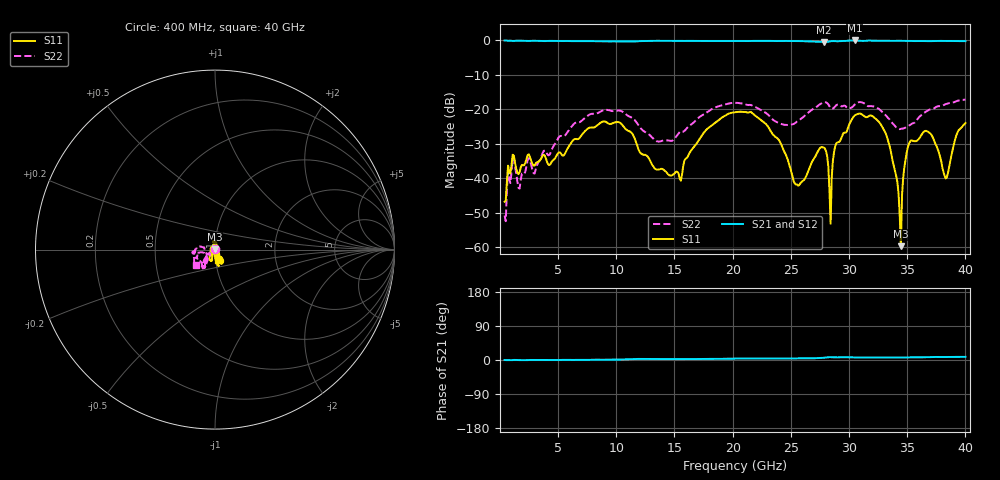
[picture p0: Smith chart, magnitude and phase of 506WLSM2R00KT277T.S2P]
!  American Technical Ceramics  Date:  8/31/2012
!  One Norden Lane
!  Huntington Station,  NY.  11746-2102
!  Tel:  (631) 622-4700  Fax:  (631) 622-4748
!  Part Number  506WLSM2R00KT277T
!  Description:  Ultra-Broadband Inductor
!  Application:  Ultra-broadband DC block decoupling, bias tee
# GHZ S DB R 50
! Freq  |S11|  S11 Ph  |S21|  S21 Ph  |S12|  S12 Ph  |S22|  S22 Ph
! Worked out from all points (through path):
!   401 points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, 400 MHz to 40 GHz, reference 50 ohm
!   highest |S21| = 0.00 dB at 30.5 GHz (marker M1); lowest = -0.5 dB at 27.82 GHz (marker M2)
!   lowest |S11| = -59.7 dB at 34.46 GHz (marker M3), VSWR 1.00, Z = 49.9 + j0.0755 ohm
!   |S11| at or under -10 dB: start of sweep to end of sweep
!   |S22| runs from -52.4 to -17.2 dB; largest |S21 - S12| = 0.0031
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0.4  -46.76 154.5  -0.01 -0.0  -0.01 -0.0  -50.76 132.2
1.192  -33.39 149.7  -0.14 0.2  -0.14 0.2  -34.17 153.8
1.687  -38.20 161.9  -0.06 -0.3  -0.06 -0.3  -42.96 168.4
7.033  -27.40 -110.6  -0.18 0.4  -0.18 0.5  -23.28 -126.0
10.201  -23.70 -115.8  -0.31 1.1  -0.31 1.2  -20.29 -123.8
13.666  -37.43 -140.0  -0.10 2.4  -0.10 2.5  -29.33 -139.6
15.448  -40.08 -137.4  -0.10 2.2  -0.10 2.2  -26.56 -148.8
17.626  -26.30 -88.2  -0.16 2.7  -0.16 2.8  -21.20 -135.6
20.2  -20.79 -78.7  -0.17 3.6  -0.17 3.7  -18.07 -123.6
22.873  -24.27 -80.6  -0.12 4.0  -0.12 4.0  -21.07 -124.0
25.447  -41.80 -91.1  -0.18 4.3  -0.19 4.3  -23.75 -164.1
26.833  -35.08 -123.4  -0.32 4.3  -0.31 4.4  -20.03 -170.0
27.823  -31.03 -149.9  -0.46 5.9  -0.47 5.9  -17.93 -171.4
28.417  -53.17 -19.3  -0.23 7.4  -0.23 7.4  -19.57 -171.7
28.912  -29.81 -65.0  -0.22 6.7  -0.23 6.7  -18.74 -156.4
30.496  -21.73 -56.4  -0.00 6.5  -0.01 6.6  -18.53 -127.9
33.466  -30.36 -78.1  -0.10 6.8  -0.11 6.8  -22.84 -133.7
34.456  -59.65 133.4  -0.10 6.8  -0.10 6.9  -25.63 -159.7
35.248  -29.31 98.3  -0.14 6.9  -0.14 7.0  -24.50 172.3
36.931  -26.82 88.2  -0.19 7.6  -0.19 7.7  -20.02 171.0
38.317  -40.01 22.4  -0.16 8.0  -0.16 8.0  -18.41 -167.5
40  -23.96 -73.2  -0.20 8.4  -0.21 8.5  -17.15 -141.4
